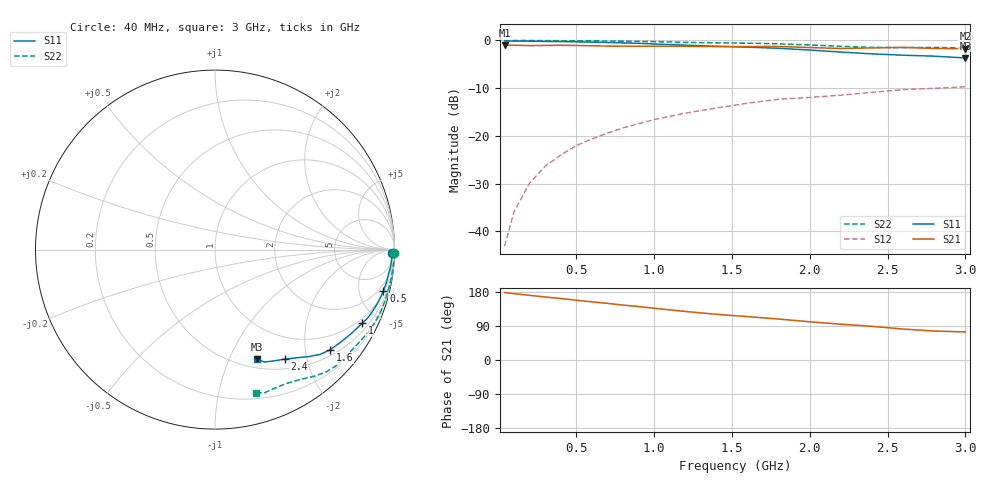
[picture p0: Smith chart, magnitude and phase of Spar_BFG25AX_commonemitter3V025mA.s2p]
! Filename:  BFG25AXG.S2P  Version:  2.0
! NXP part #: BFG25A/X  Date: May 1990
! Bias condition: Vce=3V, Ic=0.25mA
#  MHz  S  MA  R  50
! Freq  S11  S21  S12  S22  !GUM [dB]
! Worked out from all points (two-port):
!   21 points, 40 MHz to 3 GHz, reference 50 ohm
!   highest |S21| = -0.99 dB at 40 MHz (marker M1); lowest = -1.7 dB at 3 GHz (marker M2)
!   |S21| within 3 dB of the highest: start of sweep to end of sweep
!   lowest |S11| = -3.7 dB at 3 GHz (marker M3), VSWR 4.80, Z = 29.8 - j63.8 ohm
!   |S11| at or under -10 dB: nowhere
!   |S22| runs from -1.6 to 0.0 dB; largest |S21 - S12| = 0.89
!   S11 on the Smith chart (normalised r, x): 40 MHz: 51, -64; 500 MHz: 1.17, -8.10; 1 GHz: 0.79, -4.09; 1.6 GHz: 0.63, -2.53; 2.4 GHz: 0.64, -1.63; 3 GHz: 0.60, -1.28
40  0.985 -1.1  0.892 178.0  0.007 84.5  0.999 -1.2
100  0.986 -2.9  0.89 175.0  0.016 88.0  0.999 -3.0
200  0.983 -5.6  0.883 170.7  0.032 85.1  0.997 -5.9
300  0.976 -8.3  0.886 166.3  0.048 83.3  0.995 -8.9
400  0.972 -11.1  0.889 162.2  0.063 80.8  0.992 -11.8
500  0.966 -13.8  0.885 157.8  0.079 78.9  0.991 -14.8
600  0.959 -16.5  0.879 153.4  0.093 77.3  0.988 -17.6
700  0.952 -18.9  0.872 149.5  0.107 75.5  0.986 -20.4
800  0.942 -21.5  0.87 145.0  0.121 74.0  0.981 -23.0
900  0.933 -24.0  0.869 141.1  0.134 72.1  0.976 -25.6
1000  0.917 -26.6  0.869 136.6  0.148 70.1  0.97 -28.3
1200  0.892 -31.6  0.868 128.1  0.173 65.3  0.953 -33.4
1400  0.869 -36.5  0.862 120.6  0.196 62.0  0.942 -38.6
1600  0.85 -41.1  0.861 114.5  0.22 59.3  0.936 -43.6
1800  0.827 -44.9  0.864 108.1  0.242 55.9  0.921 -47.8
2000  0.793 -48.7  0.842 100.8  0.253 52.3  0.897 -51.8
2200  0.755 -53.0  0.823 94.5  0.267 49.3  0.867 -56.5
2400  0.723 -57.6  0.835 88.8  0.286 45.2  0.845 -62.0
2600  0.7 -62.5  0.845 81.7  0.305 41.3  0.841 -67.0
2800  0.684 -66.3  0.824 76.4  0.315 39.1  0.844 -70.8
3000  0.655 -68.9  0.818 74.1  0.327 39.3  0.832 -73.9
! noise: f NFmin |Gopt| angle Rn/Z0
500  1.5  0.9  4  4.2
1000  1.6  0.81  13  4
2000  1.8  0.86  37  2.4
